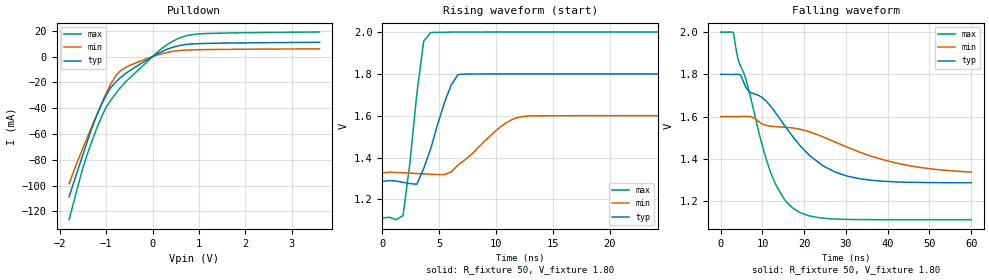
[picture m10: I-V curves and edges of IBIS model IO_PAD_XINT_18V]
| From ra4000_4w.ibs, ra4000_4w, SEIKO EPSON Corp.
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[Model]   IO_PAD_XINT_18V
Model_type Open_drain
Polarity Non-Inverting
Vref=2.00
Vmeas=0.90
Rref=5000
C_comp   2.5p   2.0p   3.0p
[Temperature Range] 25   125   -40
[Voltage Range]   1.80   1.60   2.00
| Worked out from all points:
|   slope of the pulldown table from 0 to 0.27 V, typ, clamps not added: 54.4 ohm
|   falling waveform, R_fixture 50, V_fixture 1.80: 20-80 % time 13.7ns typ, 23.5ns min, 7.76ns max; typ from 1.8 V to 1.29 V
|   rising waveform, R_fixture 50, V_fixture 1.80: 20-80 % time 1.8ns typ, 3.29ns min, 1.1ns max; typ from 1.29 V to 1.8 V
[Pulldown]
-1.8V     -108.9mA   -98.7mA    -126.5mA
-1.5V     -75.95mA   -70.76mA   -86.06mA
-1.4V     -65.08mA   -62.09mA   -75.07mA
-1.2V     -45.3mA    -45.03mA   -55.4mA
-1V       -29.91mA   -28.44mA   -39.28mA
-800mV    -19.93mA   -15.3mA    -29mA
-700mV    -16.58mA   -11.24mA   -24.44mA
-400mV    -8.853mA   -5.464mA   -13.51mA
200mV     3.863mA    2.205mA    6.265mA
600mV     8.675mA    4.737mA    14.69mA
900mV     9.873mA    5.241mA    17.26mA
3.6V      11.07mA    5.981mA    19.07mA
[Falling Waveform]
R_fixture=50
V_fixture=1.80
V_fixture_min=1.60
V_fixture_max=2.00
0s        1.8V       1.6V       2V
3.03ns    1.8V       1.6V       1.998V
4.242ns   1.801V     1.6V       1.863V
6.061ns   1.737V     1.6V       1.775V
11.52ns   1.659V     1.556V     1.36V
16.97ns   1.512V     1.547V     1.171V
24.24ns   1.37V      1.506V     1.119V
30.3ns    1.318V     1.455V     1.112V
44.85ns   1.289V     1.368V     1.111V
60ns      1.286V     1.337V     1.111V
[Rising Waveform]
R_fixture=50
V_fixture=1.80
V_fixture_min=1.60
V_fixture_max=2.00
0s        1.286V     1.326V     1.111V
1.818ns   1.281V     1.327V     1.123V
3.03ns    1.272V     1.324V     1.703V
3.636ns   1.348V     1.322V     1.956V
4.242ns   1.439V     1.32V      1.997V
5.455ns   1.662V     1.318V     1.999V
6.667ns   1.797V     1.365V     1.999V
10.91ns   1.8V       1.566V     2V
12.73ns   1.8V       1.598V     2V
60ns      1.8V       1.6V       2V
[Ramp]
R_load=50
dV/dt_r   3.085E-1/1.825E-9   1.642E-1/3.454E-9   5.334E-1/1.080E-9
dV/dt_f   3.084E-1/1.367E-8   1.579E-1/2.351E-8   5.334E-1/7.707E-9
|[End   IO_PAD_XINT_18V
